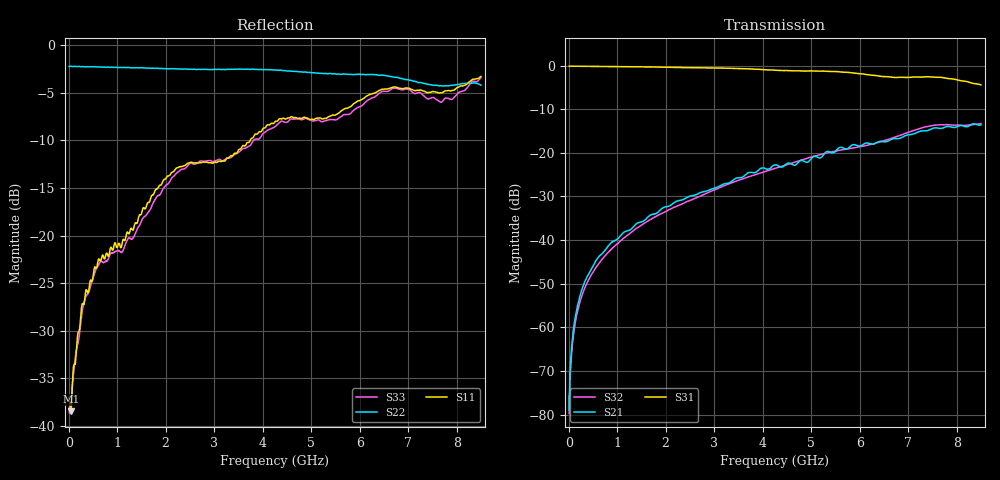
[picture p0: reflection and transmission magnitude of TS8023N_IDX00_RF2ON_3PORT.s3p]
!Created with skrf (http://scikit-rf.org).
# GHz S RI R 50.0
!freq ReS11 ImS11 ReS12 ImS12 ReS13 ImS13
! ReS21 ImS21 ReS22 ImS22 ReS23 ImS23
! ReS31 ImS31 ReS32 ImS32 ReS33 ImS33
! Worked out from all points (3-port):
!   1601 points, 10 MHz to 8.5 GHz, reference 50 ohm
!   strongest paths, dB at 10 MHz, 2.132 GHz, 4.255 GHz, 6.378 GHz, 8.5 GHz:
!     S31: -0.1, -0.4, -1.1, -2.4, -4.4
!     S21: -79.0, -31.8, -22.8, -17.5, -13.6
!     S32: -79.7, -32.7, -23.6, -17.6, -13.3
!   lowest |S11| = -38.5 dB at 47.14 MHz (marker M1), VSWR 1.02, Z = 50.9 - j0.763 ohm
!   |S11| at or under -10 dB: start of sweep to 3.743 GHz
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0.01  0.0136 -0.000307  5.56e-05 0.000102  0.9835 -0.00332
      5.88e-05 9.52e-05  -0.7732 0.00279  3.19e-05 7.61e-05
      0.9835 -0.00343  3.87e-05 9.63e-05  0.0124 0.000109
0.04714375  0.00928 -0.00749  4.39e-05 0.000436  0.9834 -0.0145
            4.16e-05 0.000467  -0.7763 0.00942  3.1e-05 0.000402
            0.9833 -0.0144  5.16e-05 0.000406  0.0107 -0.00647
0.1267375  0.00874 -0.0192  1.14e-05 0.00122  0.9815 -0.0371
           1.28e-05 0.00121  -0.7746 0.0226  2.25e-05 0.00106
           0.9813 -0.0373  3.3e-05 0.00102  0.00947 -0.0196
0.2753125  0.0102 -0.0421  -8.84e-05 0.00271  0.977 -0.0798
           -9.79e-05 0.00273  -0.7705 0.0467  -2.16e-06 0.00231
           0.9771 -0.0798  -4.16e-06 0.00234  0.00523 -0.0389
0.8643063  -0.00438 -0.086  -0.000272 0.00919  0.9443 -0.2413
           -0.000245 0.0092  -0.7487 0.1604  -7.29e-05 0.00768
           0.9443 -0.2413  -6.62e-05 0.00769  -0.0182 -0.0783
2.228013  -0.1031 -0.2015  0.002 0.028  0.7585 -0.5725
          0.00201 0.0279  -0.6456 0.3843  0.00436 0.024
          0.7585 -0.5725  0.00433 0.0241  -0.1359 -0.1638
4.255  -0.3489 -0.1882  0.0306 0.0662  0.2905 -0.8368
       0.0305 0.0662  -0.3508 0.652  0.037 0.0549
       0.2891 -0.8361  0.0372 0.055  -0.3671 -0.0658
6.764856  -0.5858 0.1356  0.1249 0.0751  -0.262 -0.683
          0.1246 0.0752  0.073 0.6737  0.1488 0.0396
          -0.2615 -0.6818  0.1491 0.0392  -0.5018 0.3155
7.677531  -0.5004 0.2565  0.1846 0.0476  -0.4269 -0.5957
          0.1845 0.0477  0.2838 0.5429  0.2067 -0.0363
          -0.4257 -0.5946  0.2068 -0.0368  -0.2657 0.425
8.5  -0.4956 0.4736  0.2094 0.0114  -0.4731 -0.3686
     0.2097 0.0115  0.3596 0.5011  0.2011 -0.0821
     -0.4729 -0.369  0.2009 -0.082  -0.1173 0.6648
